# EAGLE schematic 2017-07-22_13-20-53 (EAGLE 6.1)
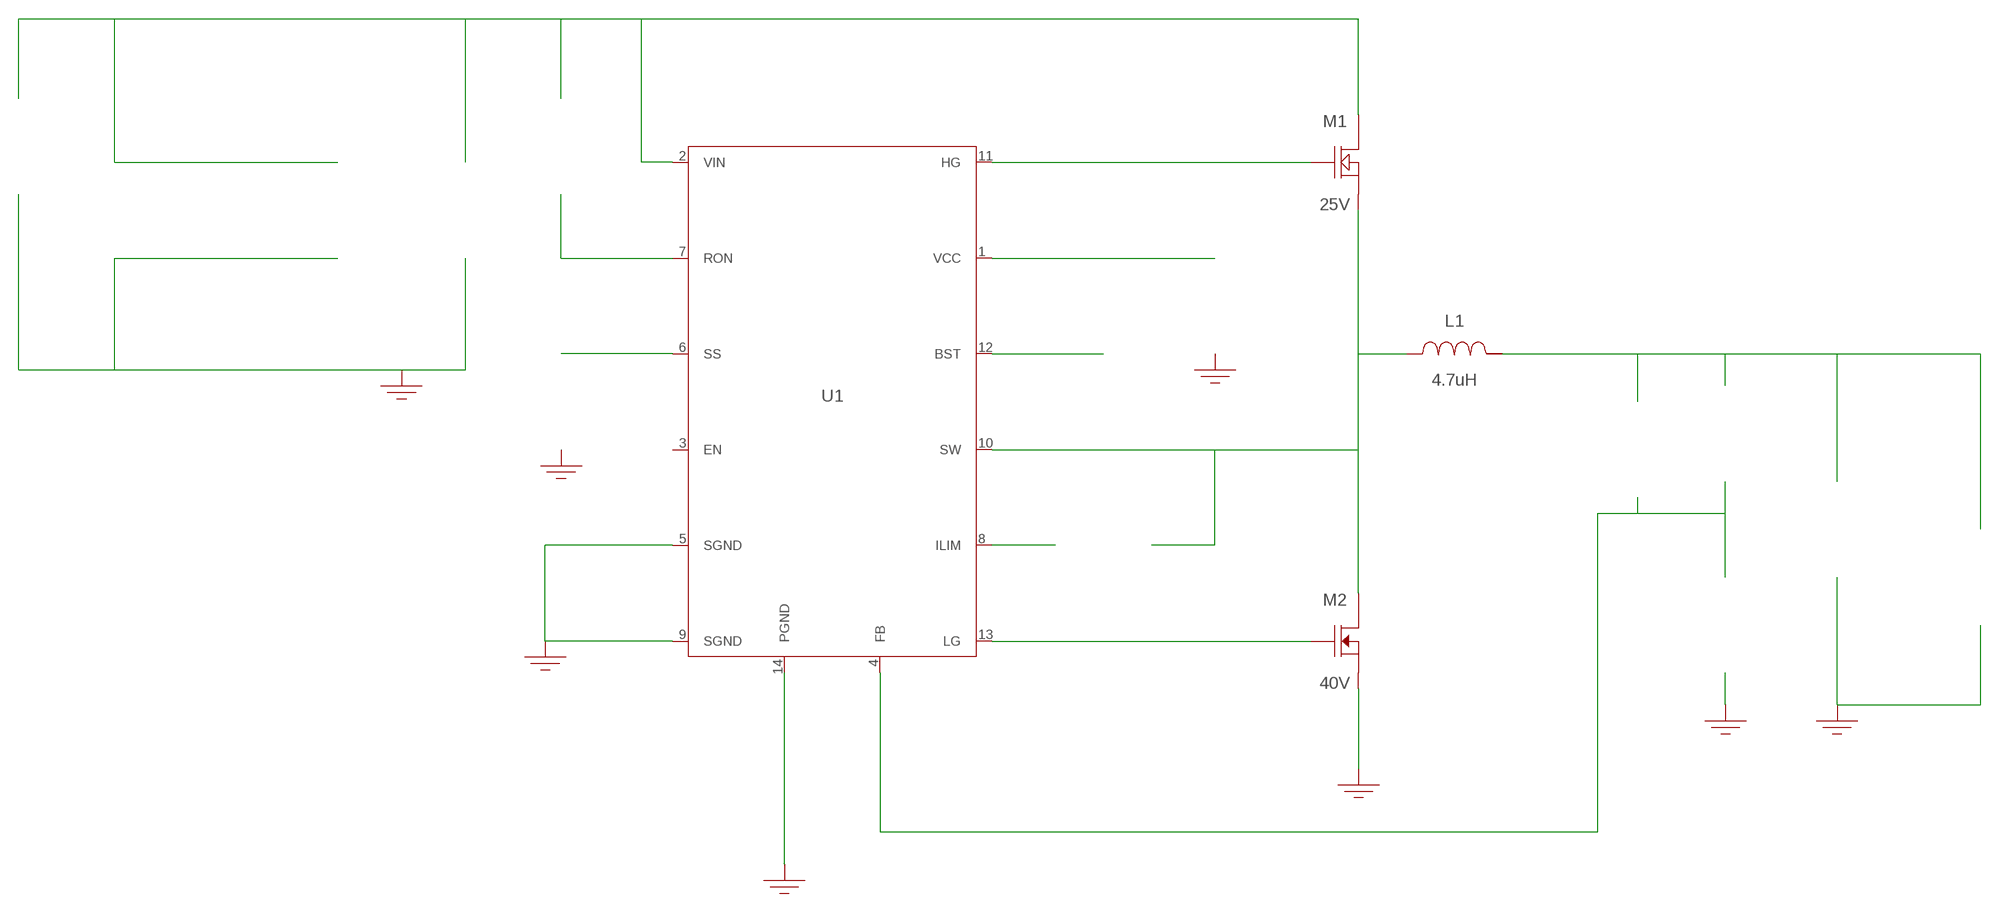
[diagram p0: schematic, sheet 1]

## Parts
CBST  470nF  EMK212B7474KD-TEMK212B7474KD-T  [0805]  (not placed on a sheet)
CBYP  100nF  08053C104KAT2A08053C104KAT2A  [0805]  (not placed on a sheet)
CFF  1nF  C0805C102K5RACTUC0805C102K5RACTU  [0805]  (not placed on a sheet)
CIN  47uF  C3216X5R1E476M160ACC3216X5R1E476M160AC  [1206]  (not placed on a sheet)
CIN_2  47uF  C3216X5R1E476M160ACC3216X5R1E476M160AC  [1206]  (not placed on a sheet)
CIN_3  47uF  C3216X5R1E476M160ACC3216X5R1E476M160AC  [1206]  (not placed on a sheet)
COUT  330uF  6SVPC330M6SVPC330M  [SM_RADIAL_6.3AMM]  (not placed on a sheet)
CSS  15nF  CC0805KRX7R9BB153CC0805KRX7R9BB153  [0805]  (not placed on a sheet)
CVCC  1uF  EMK212B7105KG-TEMK212B7105KG-T  [0805]  (not placed on a sheet)
GND1  WB_GND  WB_GNDWB_GND  [WB_GND]
GND2  WB_GND  WB_GNDWB_GND  [WB_GND]
GND3  WB_GND  WB_GNDWB_GND  [WB_GND]
GND4  WB_GND  WB_GNDWB_GND  [WB_GND]
GND5  WB_GND  WB_GNDWB_GND  [WB_GND]
GND6  WB_GND  WB_GNDWB_GND  [WB_GND]
GND7  WB_GND  WB_GNDWB_GND  [WB_GND]
GND8  WB_GND  WB_GNDWB_GND  [WB_GND]
IOUT_1  WB_CURRENT_LOAD  WB_CURRENT_LOADWB_CURRENT_LOAD  [WB_CURRENT_LOAD]  (not placed on a sheet)
L1  4.7uH  XAL1010-472MEBXAL1010-472MEB  [XAL1010]
M1  25V  CSD16321Q5CSD16321Q5  [TRANS_NexFET_Q5]
M2  40V  CSD18509Q5BCSD18509Q5B  [TRANS_NexFET_Q5B]
RFB1  10k  ERJ-6ENF1002VERJ-6ENF1002V  [0805]  (not placed on a sheet)
RFB2  73.2k  ERJ-6ENF7322VERJ-6ENF7322V  [0805]  (not placed on a sheet)
RILIM  464  CRCW0805464RFKEACRCW0805464RFKEA  [0805]  (not placed on a sheet)
RON  237k  ERJ-6ENF2373VERJ-6ENF2373V  [0805]  (not placed on a sheet)
U1  LM3150MH/NOPB  LM3150MH/NOPBLM3150MH/NOPB  [MXA14A]
VIN  WB_BATTERY  WB_BATTERYWB_BATTERY  [WB_BATTERY]  (not placed on a sheet)

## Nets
0: Cbyp.2@2 Cin.2@2 Cin_2.2@2 Cin_3.2@2 Cout.-@2 Css.2@2 Cvcc.2@2 GND1.1 GND2.1 GND3.1 GND4.1 GND5.1 GND6.1 GND7.1 GND8.1 Iout_1.-@2 M2.1(Source) M2.2(Source) M2.3(Source) Rfb1.2@2 U1.5(SGND) U1.9(SGND) U1.14(PGND) U1.15(DAP) Vin.-@2
1: Css.1@1 U1.6(SS)
2: Cbyp.1@1 Cin.1@1 Cin_2.1@1 Cin_3.1@1 M1.5(Drain) M1.6(Drain) M1.7(Drain) M1.8(Drain) M1.9(Drain) Ron.1@1 U1.2(VIN) Vin.+@1
3: Ron.2@2 U1.7(RON)
4: Cff.1@1 Cout.+@1 Iout_1.+@1 L1.2 Rfb2.1@1
5: Cff.2@2 Rfb1.1@1 Rfb2.2@2 U1.4(FB)
6: Cbst.2@2 L1.1 M1.1(Source) M1.2(Source) M1.3(Source) M2.5(Drain) M2.6(Drain) M2.7(Drain) M2.8(Drain) M2.9(Drain) Rilim.1@1 U1.10(SW)
7: M2.4(Gate) U1.13(LG)
8: M1.4(Gate) U1.11(HG)
9: Cbst.1@1 U1.12(BST)
10: Cvcc.1@1 U1.1(VCC)
11: Rilim.2@2 U1.8(ILIM)
Unconnected: CBST.1 CBST.2 CBYP.1 CBYP.2 CFF.1 CFF.2 CIN.1 CIN.2 CIN_2.1 CIN_2.2 CIN_3.1 CIN_3.2 COUT.1(+) COUT.2(-) CSS.1 CSS.2 CVCC.1 CVCC.2 IOUT_1.1(+) IOUT_1.2(-) RFB1.1 RFB1.2 RFB2.1 RFB2.2 RILIM.1 RILIM.2 RON.1 RON.2 U1.3(EN) VIN.1(+) VIN.2(-)

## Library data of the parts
CBST = AcceleratedDesigns_Lib:EMK212B7474KD-T; Cap: 4.7E-7; ESR: 0.0; IRMS: 0.0; Manufacturer_Name: Taiyo Yuden; Manufacturer_Part_Number: EMK212B7474KD-T; VDC: 16.0; Vendor: Taiyo Yuden
CBYP = AcceleratedDesigns_Lib:08053C104KAT2A; Cap: 1.0E-7; ESR: 0.28; IRMS: 0.0; Manufacturer_Name: AVX; Manufacturer_Part_Number: 08053C104KAT2A; VDC: 25.0; Vendor: AVX
CFF = AcceleratedDesigns_Lib:C0805C102K5RACTU; Cap: 1.0E-9; ESR: 0.384; IRMS: 0.214; Manufacturer_Name: Kemet; Manufacturer_Part_Number: C0805C102K5RACTU; VDC: 50.0; Vendor: Kemet
CIN CIN_2 CIN_3 = AcceleratedDesigns_Lib:C3216X5R1E476M160AC; Cap_F: 0.000047; Manufacturer_Name: TDK; Manufacturer_Part_Number: C3216X5R1E476M160AC; MountType: SMT; RoHS: Y; VDC_V: 25
COUT = AcceleratedDesigns_Lib:6SVPC330M; Cap: 3.3E-4; Datasheet_URL: https://industrial.panasonic.com/content/data/CP/PDF/OS%2DCON/S%5FOS%2DCON%5FSVPC%5Fe.pdf; ESR: 0.017; IRMS: 3.39; Manufacturer_Name: Panasonic; Manufacturer_Part_Number: 6SVPC330M; VDC: 6.3; Vendor: Panasonic
CSS = AcceleratedDesigns_Lib:CC0805KRX7R9BB153; Cap: 1.5E-8; ESR: 0.0; IRMS: 0.0; Manufacturer_Name: Yageo America; Manufacturer_Part_Number: CC0805KRX7R9BB153; VDC: 50.0; Vendor: Yageo America
CVCC = AcceleratedDesigns_Lib:EMK212B7105KG-T; Cap: 1.0E-6; ESR: 0.0; IRMS: 0.0; Manufacturer_Name: Taiyo Yuden; Manufacturer_Part_Number: EMK212B7105KG-T; VDC: 16.0; Vendor: Taiyo Yuden
GND1-GND8 = AcceleratedDesigns_Lib:WB_GND; Manufacturer_Name: WB_GND; Manufacturer_Part_Number: WB_GND; PowerPortType: POWER_GROUND; Value: Value
IOUT_1 = AcceleratedDesigns_Lib:WB_CURRENT_LOAD; Manufacturer_Name: WB_CURRENT_LOAD; Manufacturer_Part_Number: WB_CURRENT_LOAD; PowerPortType: POWER_GROUND; Value: Value
L1 = AcceleratedDesigns_Lib:XAL1010-472MEB; DCR: 0.01; IDC: 24.0; L: 4.7E-6; Manufacturer_Name: Coilcraft; Manufacturer_Part_Number: XAL1010-472MEB; Vendor: Coilcraft
M1 = AcceleratedDesigns_Lib:CSD16321Q5; Datasheet_URL: http://www.ti.com/lit/ds/symlink/csd16321q5.pdf; IdsMax: 100.0; Manufacturer_Name: Texas Instruments; Manufacturer_Part_Number: CSD16321Q5; QgTyp: 14.0; Quantity: 1; Rdson45: 0.0021; VdsMax: 25.0; Vendor: Texas Instruments
M2 = AcceleratedDesigns_Lib:CSD18509Q5B; Datasheet_URL: http://www.ti.com/lit/ds/symlink/csd18502Q5B.pdf; IdsMax: 100.0; Manufacturer_Name: Texas Instruments; Manufacturer_Part_Number: CSD18509Q5B; QgTyp: 25.0; Quantity: 1; Rdson45: 0.0033; VdsMax: 40.0; Vendor: Texas Instruments
RFB1 = AcceleratedDesigns_Lib:ERJ-6ENF1002V; Manufacturer_Name: Panasonic; Manufacturer_Part_Number: ERJ-6ENF1002V; Power: 0.125; Resistance: 10000.0; Tolerance: 1.0; Vendor: Panasonic
RFB2 = AcceleratedDesigns_Lib:ERJ-6ENF7322V; Manufacturer_Name: Panasonic; Manufacturer_Part_Number: ERJ-6ENF7322V; Power: 0.125; Resistance: 73200.0; Tolerance: 1.0; Vendor: Panasonic
RILIM = AcceleratedDesigns_Lib:CRCW0805464RFKEA; Manufacturer_Name: Vishay-Dale; Manufacturer_Part_Number: CRCW0805464RFKEA; Power: 0.125; Resistance: 464.0; Tolerance: 1.0; Vendor: Vishay-Dale
RON = AcceleratedDesigns_Lib:ERJ-6ENF2373V; Manufacturer_Name: Panasonic; Manufacturer_Part_Number: ERJ-6ENF2373V; Power: 0.125; Resistance: 237000.0; Tolerance: 1.0; Vendor: Panasonic
U1 = AcceleratedDesigns_Lib:LM3150MH/NOPB; Datasheet_URL: http://www.ti.com/product/lm3150; Frequency: 1000000.0; Imax: 12.0; Manufacturer_Name: Texas Instruments; Manufacturer_Part_Number: LM3150MH/NOPB; Mktg_Package: NA; NSID: LM3150MH/NOPB; Package: NA; Vendor: Texas Instruments
VIN = AcceleratedDesigns_Lib:WB_BATTERY; Manufacturer_Name: WB_BATTERY; Manufacturer_Part_Number: WB_BATTERY; PowerPortType: POWER_GROUND; Value: Value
